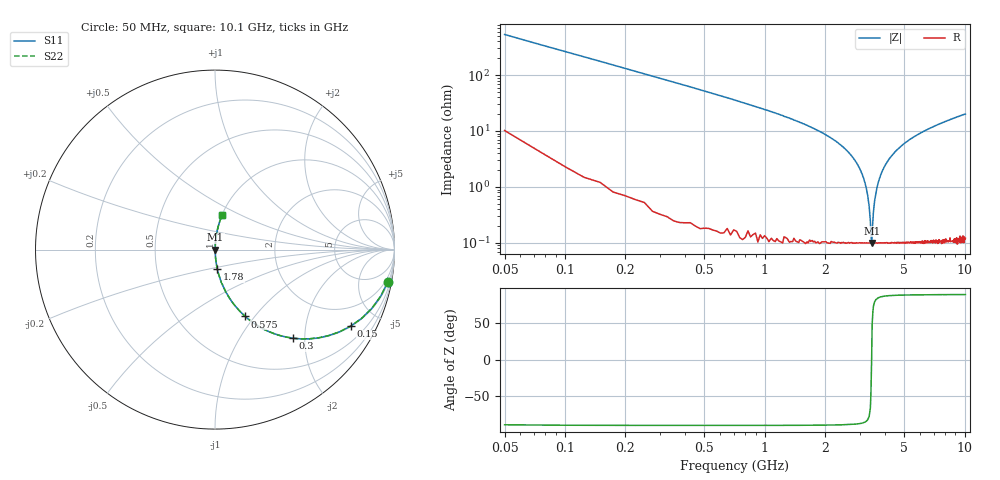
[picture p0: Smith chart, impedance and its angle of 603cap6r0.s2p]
! AVX Thin Film Operation		Date: November 2004
! Description: Accu-P® Series, Thin Film, SMD, RF Capacitor
! Part Number: 06035J6R0BBT
! 50 MHz  -  10.05 GHz
! Serial Measurements
# hz S db R 50
!	S11		S21		S12		S22
!	dB	Phase	dB	Phase	dB	Phase	dB	Phase
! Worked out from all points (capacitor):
!   400 points, 50 MHz to 10.1 GHz, reference 50 ohm
!   read as one part in series: C = 6 pF near 100 MHz
!   lowest |Z| = 100 mohm at 3.43 GHz (marker M1)
!   series resonance near 3.429 GHz, so ESL is about 360 pH
!   S11 on the Smith chart (normalised r, x): 50 MHz: 1, -11; 150 MHz: 1.02, -3.54; 300 MHz: 1.01, -1.76; 575 MHz: 1.00, -0.90; 1.78 GHz: 1.00, -0.22; 10.1 GHz: 1.00, +0.40
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5e7  -0.18 -10.6  -14.70 78.3  -14.70 78.3  -0.18 -10.6
1e8  -0.60 -20.6  -9.07 68.9  -9.07 68.9  -0.60 -20.6
1.5e8  -1.23 -29.4  -6.17 60.2  -6.17 60.2  -1.23 -29.4
3e8  -3.63 -48.6  -2.50 41.2  -2.50 41.2  -3.63 -48.6
5.75e8  -7.78 -65.7  -0.81 24.1  -0.81 24.1  -7.78 -65.7
1.73e9  -18.90 -82.9  -0.07 6.5  -0.07 6.5  -18.90 -82.9
1.78e9  -19.30 -83.2  -0.06 6.2  -0.06 6.2  -19.30 -83.2
2.53e9  -26.40 -86.1  -0.02 2.7  -0.02 2.7  -26.40 -86.1
3.03e9  -34.30 -85.9  -0.01 1.1  -0.01 1.1  -34.30 -85.9
3.28e9  -43.10 -81.4  -0.01 0.4  -0.01 0.4  -43.10 -81.4
3.33e9  -46.60 -77.4  -0.01 0.3  -0.01 0.3  -46.60 -77.4
3.38e9  -52.20 -65.9  -0.01 0.1  -0.01 0.1  -52.20 -65.9
3.4e9  -56.50 -47.9  -0.01 0.1  -0.01 0.1  -56.50 -47.9
3.43e9  -60.00 1.4  -0.01 -0.0  -0.01 -0.0  -60.00 1.4
3.5e9  -49.10 73.3  -0.01 -0.2  -0.01 -0.2  -49.10 73.3
3.55e9  -44.90 79.5  -0.01 -0.3  -0.01 -0.3  -44.90 79.5
3.8e9  -35.80 85.5  -0.01 -0.9  -0.01 -0.9  -35.80 85.5
4.2e9  -29.90 86.4  -0.01 -1.8  -0.01 -1.8  -29.90 86.4
5.08e9  -24.10 85.5  -0.03 -3.6  -0.03 -3.6  -24.10 85.5
6.75e9  -19.00 83.0  -0.06 -6.5  -0.06 -6.5  -19.00 83.0
8.43e9  -16.10 80.6  -0.12 -9.0  -0.12 -9.0  -16.10 80.6
1.01e10  -14.10 78.3  -0.18 -11.3  -0.18 -11.3  -14.10 78.3
